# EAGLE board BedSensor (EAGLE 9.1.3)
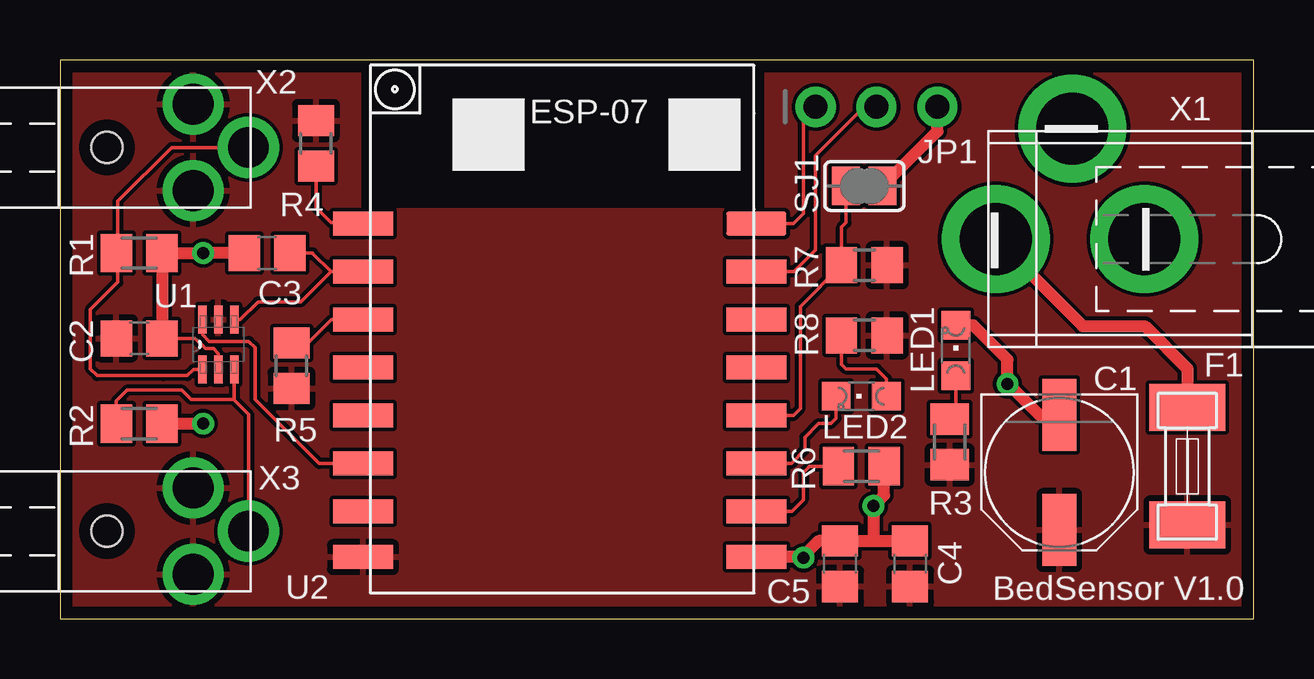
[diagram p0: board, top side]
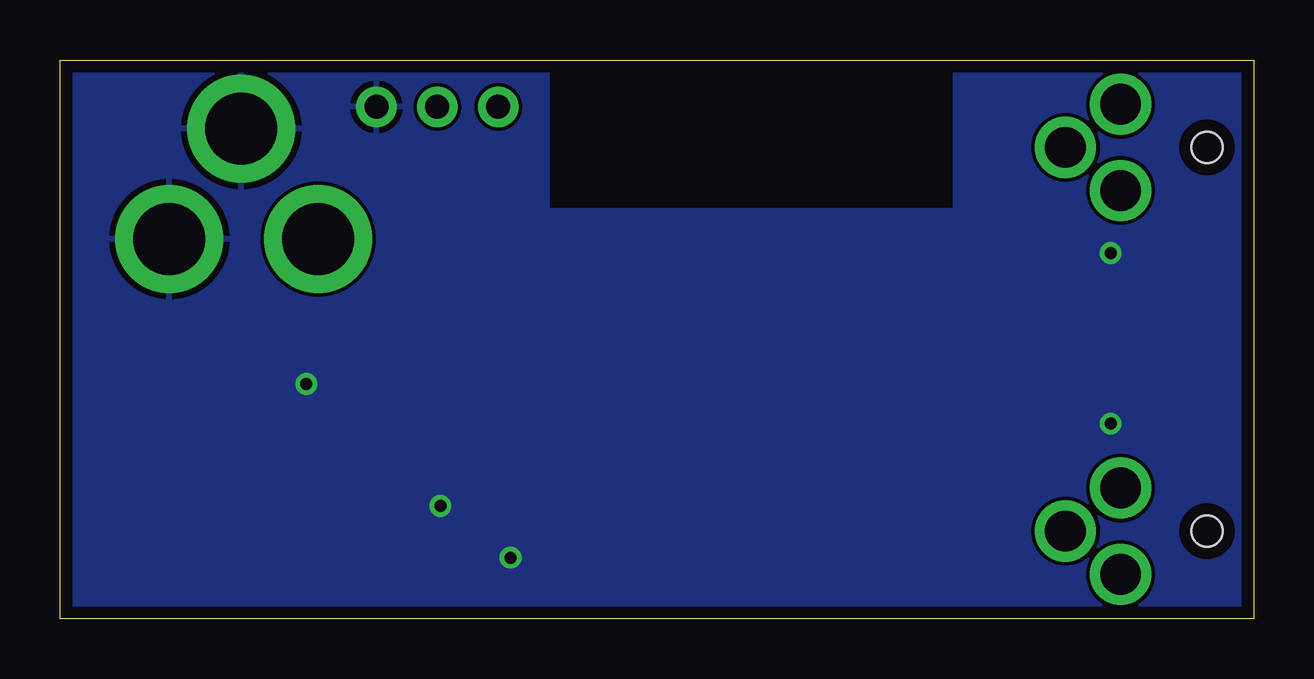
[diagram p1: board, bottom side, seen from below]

Size 49.76 x 23.29 mm. Coordinates in mm from the lower left corner, seen from the top.
Outline: 0,0 48.26,0 49.76,0 49.76,23.29 0,23.29 0,22.86 0,0
Copper layers (1*16): Top 0.035mm / dielectric 1.5mm / Bottom 0.035mm
Design rules "default *": minimum track width 6mil, minimum drill 0.35mm, track to track 6mil, track to pad 6mil, pad to pad 6mil, via to via 6mil, smd to smd 6mil, copper to edge 20mil, drill to drill 6mil, minimum pad ring 10mil, minimum via ring 8mil, stop-mask expansion 4mil, vias tented up to drill 0mil, thermal gap 10mil
tRestrict: area 12.6,17.1 to 29.3,23.2
bRestrict: area 12.6,17.1 to 29.3,23.2

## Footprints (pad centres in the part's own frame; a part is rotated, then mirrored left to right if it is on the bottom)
PANASONIC_D = smd 3 x 1.4: + 2.4,0; - -2.4,0
C0805 = smd 1.3 x 1.5: 1 -0.95,0; 2 0.95,0
SMD-6,1X2,6 = smd 1.96 x 3.15: 1 -2.45,0; 2 2.45,0
1X03_ROUND = drill 1 pad 1.676: 1 -2.54,0; 2 0,0; 3 2.54,0
CHIPLED_0805 = smd 1.2 x 1.2: A 0,-1.05; C 0,1.05
M0805 = smd 1.3 x 1.6: 1 -0.95,0; 2 0.95,0
R0805 = smd 1.3 x 1.5: 1 -0.95,0; 2 0.95,0
SJ = smd 1.168 x 1.6: 1 -0.762,0; 2 0.762,0
SOT65P210X110-6N = smd 1.168 x 0.356: 1 -1.041,0.66; 2 -1.041,0; 3 -1.041,-0.66; 4 1.041,-0.66; 5 1.041,0; 6 1.041,0.66
ESP07-16PIN = smd 2.5 x 1: ADC -8.2,3.8; CH_PD -8.2,1.8; GND 8.2,-8.105; GPIO0 8.2,-2.2; GPIO2 8.2,-4.2; GPIO4 8.2,1.8; GPIO5 8.2,-0.2; GPIO12 -8.2,-4.2; GPIO13 -8.2,-6.2; GPIO14 -8.2,-2.2; GPIO15 8.2,-6.2; GPIO16 -8.2,-0.2; REST -8.2,5.8; RX 8.2,3.8; TX 8.2,5.8; VCC -8.2,-8.105
HEBW21 = drill 3 pad 4.5: 1 7.5,4.5; 2 10.5,-0.1; 3 13.7,4.5
JY029 = drill 1.7: P$1 10.9,2.5; P$2 8.6,0.7; P$3 8.6,4.3 | hole 1.3: 5,2.5

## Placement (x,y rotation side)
C1  100u/16V  [PANASONIC_D]  41.66,6.1 270 top
C2  100n  [C0805]  3.3,11.68 0 top
C3  10n  [C0805]  8.64,15.24 180 top
C4  100n  [C0805]  35.43,2.29 90 top
C5  10u  [C0805]  32.51,2.29 90 top
F1  T500mA  [SMD-6,1X2,6]  46.99,6.35 270 top
JP1  [1X03_ROUND]  34.04,21.34 0 top
LED1  GREEN  [CHIPLED_0805]  37.34,11.18 0 top
LED2  YELLOW  [CHIPLED_0805]  33.4,9.27 90 top
R1  100  [M0805]  3.3,15.24 180 top
R2  100  [M0805]  3.3,8.13 180 top
R3  330  [M0805]  37.08,7.37 270 top
R4  10K  [R0805]  10.67,19.81 270 top
R5  10K  [R0805]  9.65,10.54 90 top
R6  10k  [M0805]  33.4,6.35 0 top
R7  10K  [R0805]  33.53,14.73 0 top
R8  330  [R0805]  33.53,11.81 0 top
SJ1  [SJ]  33.53,18.03 180 top
U1  SN74LVC1G3157DCKR  [SOT65P210X110-6N]  6.6,11.43 90 top
U2  ESP07-16PIN  [ESP07-16PIN]  20.83,10.67 0 top
X1  HEBW21  [HEBW21]  52.7,20.32 180 top
X2  JY029  [JY029]  -3.05,17.14 0 top
X3  JY029  [JY029]  -3.05,1.14 0 top

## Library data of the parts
C1-C5 = rcl; SPICEPREFIX: C
F1 = f-lf-omniblok-s
JP1 = microbuilder
LED1 LED2 = led
R1-R8 = rcl; SPICEPREFIX: R
SJ1 = jumper
U1 = SN74LVC1G3157DCKR; AVAILABILITY: Good; DESCRIPTION: Single-Pole, Double-Throw Analog Switch 6-SC70 -40 to 85; MF: Texas Instruments; MP: SN74LVC1G3157DCKR; PACKAGE: SC-70 Texas Instruments; PRICE: 0.12 USD
U2 = esp8266modules; DIMENSIONS: 22.0 x 16.0 mm; PINS: 16; PITCH: 0.078" / 2 mm
X1-X3 = con-jack

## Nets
+3V3: C1.+ C2.1 C4.1 C5.1 F1.2 R3.2 R4.1 R5.1 R7.2 R8.2 U1.5 U2.VCC X2.P$2 X2.P$3 X3.P$2 X3.P$3
GND: C1.- C2.2 C3.2 C4.2 C5.2 JP1.3 LED1.C R1.1 R2.1 R6.2 SJ1.1 U1.2 U2.GND X1.1 X1.2
N$1: LED1.A R3.1
N$2: JP1.1 U2.TX
N$3: F1.1 X1.3
N$5: R1.2 U1.1 X2.P$1
N$6: R6.1 U2.GPIO15
N$7: C3.1 U1.4 U2.ADC
N$9: R2.2 U1.3 X3.P$1
N$11: JP1.2 U2.RX
N$12: R7.1 SJ1.2 U2.GPIO0
N$13: LED2.C U2.GPIO2
N$14: U1.6 U2.GPIO12
N$15: R4.2 U2.REST
N$16: R5.2 U2.CH_PD
N$17: LED2.A R8.1

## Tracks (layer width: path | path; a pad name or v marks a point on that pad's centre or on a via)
+3V3
  pour Top: 0,23.24 49.78,23.24 49.78,0 0,0
GND  (via drill 0.5)
  Top 0.152: U1.2 6.6,11.05 6.4,11.25 6.08,11.25 5.65,11.68 C2.2
  Top 0.5: C3.2 v5.97,15.24 R1.1 C2.2 | R2.1 v5.97,8.13 | 34.04,3.24 C5.2 31.62,3.24 30.95,2.56 U2.GND | 34.04,3.24 C4.2 | 34.04,3.24 33.91,3.36 v33.91,4.7 34.35,5.14 R6.2 | SJ1.1 36.58,20.32 JP1.3 | C1.- 40.81,8.5 39.53,9.78 v39.5,9.78 39.5,10.79 38.07,12.23 LED1.C
  other vias: 30.99,2.54
  pour Bottom: 0,23.24 49.78,23.24 49.78,0 0,0
N$1
  Top 0.152: LED1.A 37.34,8.57 R3.1
N$2
  Top 0.152: U2.TX 30.57,16.47 30.99,16.89 30.99,20.83 JP1.1
N$3
  Top 0.5: X1.3 42.63,12.19 45.21,12.19 46.99,10.41 F1.1
N$5
  Top 0.152: X2.P$1 4.66,19.64 2.41,17.4 2.41,15.24 R1.2 | U1.1 5.56,10.39 5.31,10.13 4.32,10.13 1.55,10.13 1.27,10.41 1.27,12.89 2.41,14.03 2.41,15.18 | 2.41,15.18 R1.2 | 2.41,15.18 R1.2
N$6
  Top 0.152: R6.1 31.24,6.35 30.99,6.1 30.99,4.95 30.5,4.47 U2.GPIO15
N$7
  Top 0.152: U2.ADC 11.29,14.47 | 11.29,14.47 10.03,13.21 8.26,13.21 7.52,12.47 U1.4 | 11.29,14.47 10.54,15.22 10.54,15.24 C3.1
N$9
  Top 0.152: U1.3 7.26,9.17 7.24,9.14 | 7.24,9.14 5.46,9.14 5.08,9.53 2.79,9.53 2.41,9.14 2.35,9.08 R2.2 | 7.24,9.14 7.87,8.51 7.87,3.67 X3.P$1
N$11
  Top 0.152: U2.RX 30.6,14.47 31.5,15.37 31.5,19.3 33.53,21.34 JP1.2
N$12
  Top 0.152: U2.GPIO0 30.57,8.47 30.86,8.76 30.86,13.02 R7.1 32.58,16.32 32.77,16.51 SJ1.2
N$13
  Top 0.152: 30.07,6.48 U2.GPIO2 | 30.07,6.48 | 30.07,6.48 30.48,6.48 31.05,7.05 31.05,7.56 31.62,8.13 32.13,8.13 32.35,8.35 LED2.C
N$14
  Top 0.152: U1.6 5.94,11.84 6.22,11.56 7.87,11.56 8.13,11.3 8.13,9.14 10.8,6.47 U2.GPIO12
N$15
  Top 0.152: U2.REST 12.58,16.52 12.57,16.51 11.3,16.51 10.67,17.14 R4.2
N$16
  Top 0.152: U2.CH_PD 11.32,12.47 10.79,11.94 10.35,11.49 R5.2
N$17
  Top 0.152: R8.1 32.58,10.6 32.77,10.41 34.04,10.41 34.45,10 LED2.A

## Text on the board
tNames: BedSensor V1.0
